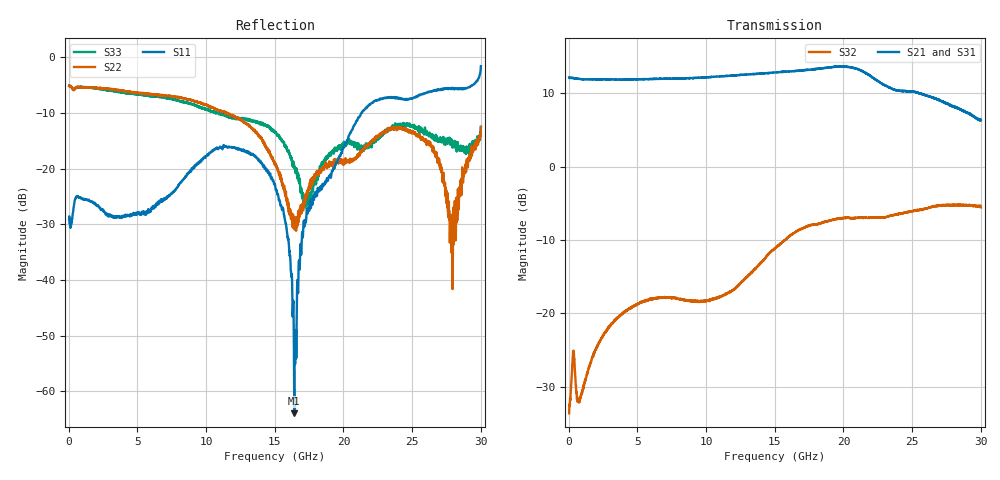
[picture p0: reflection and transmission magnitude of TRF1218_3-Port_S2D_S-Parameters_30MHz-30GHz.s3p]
! Version: APL (May 2026)
! Frequency: 30MHz to 30GHz
! Test conditions: 5V supply, T = 25
! Load conditions: 50ohm single-ended source, 50ohm diff load
! port 1 = INP, port 2 = OUTP, port 3 = OUTM
! Port[1] = INP
! Port[2] = OUTP
! Port[3] = OUTM
# hz S ri R 50
! 3 Port Network Data from SP1.SP block
! freq  reS11  imS11  reS12  imS12  reS13  imS13
!  reS21  imS21
!  reS22  imS22  reS23  imS23
!  reS31  imS31  reS32  imS32
!  reS33  imS33
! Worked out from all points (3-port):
!   2998 points, 30 MHz to 30 GHz, reference 50 ohm
!   strongest paths, dB at 30 MHz, 7.52 GHz, 15.02 GHz, 22.51 GHz, 30 GHz:
!     S21: 12.2, 12.0, 12.9, 11.7, 6.3
!     S31: 12.2, 12.0, 12.8, 11.4, 6.8
!     S32: -33.6, -17.8, -11.1, -6.9, -5.5
!   lowest |S11| = -63.9 dB at 16.42 GHz (marker M1), VSWR 1.00, Z = 50 + j0.0414 ohm
!   |S11| at or under -10 dB: start of sweep to 21.29 GHz
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3e7  -0.0341 -0.0096  0.00303 9.01e-05  0.00337 0.00139
     4.068 0.0159  -0.5601 -0.00767  0.0243 0.0072
     -4.057 -0.0357  0.0201 0.00557  -0.5586 -0.0145
4.25e9  -0.00602 -0.0378  0.00546 0.000253  0.00419 -0.00169
        0.0568 -3.93  -0.4515 0.2047  0.0524 0.061
        0.0176 3.926  0.0817 0.0657  -0.4136 0.2493
8.48e9  -0.0747 -0.0403  0.00929 -0.00277  0.00481 -0.00324
        -4.013 -0.0893  -0.2539 0.3419  0.1196 0.0982
        4.017 -0.0247  0.1152 0.0423  -0.2502 0.3032
1.209e10  -0.1477 -0.0445  0.00707 -0.00819  0.00231 -0.00531
          -0.94 4.104  0.00635 0.2953  0.2134 0.0804
          0.7327 -4.149  0.1163 0.0891  -0.0756 0.274
1.502e10  -0.071 -0.00663  0.00448 -0.0122  0.00122 -0.00672
          3.544 2.601  0.0274 0.1071  0.2349 0.0317
          -3.689 -2.359  0.2309 0.155  0.0253 0.21
1.642e10  -0.000483 0.000415  0.00165 -0.0149  -0.000129 -0.00812
          4.483 0.2783  -0.0148 0.0264  0.2366 0.0266
          -4.496 0.052  0.3299 0.1337  0.0502 0.0885
1.965e10  0.1043 -0.0691  -0.00749 -0.0125  -0.0042 -0.00653
          0.9626 -4.718  -0.1117 0.000712  0.347 0.0352
          -0.4832 4.724  0.4393 -0.0701  -0.0271 -0.1522
2.207e10  0.2312 -0.3157  -0.0107 -0.00796  -0.0074 -0.00552
          -3.518 -2.078  -0.1557 0.0882  0.4865 -0.1174
          3.598 1.672  0.4004 -0.2077  -0.1611 -0.024
2.618e10  0.014 -0.4931  -0.0109 -0.00104  -0.00511 0.00151
          -1.145 2.8  -0.161 0.0666  0.2904 -0.4775
          0.8947 -2.923  0.3063 -0.4278  -0.0753 0.1936
3e10  -0.4666 -0.6923  -0.0152 -0.00262  -0.0111 -0.000197
      1.923 0.7715  0.2313 0.0463  -0.0412 -0.5202
      -2.15 -0.4505  -0.0221 -0.5283  0.2235 0.0853
